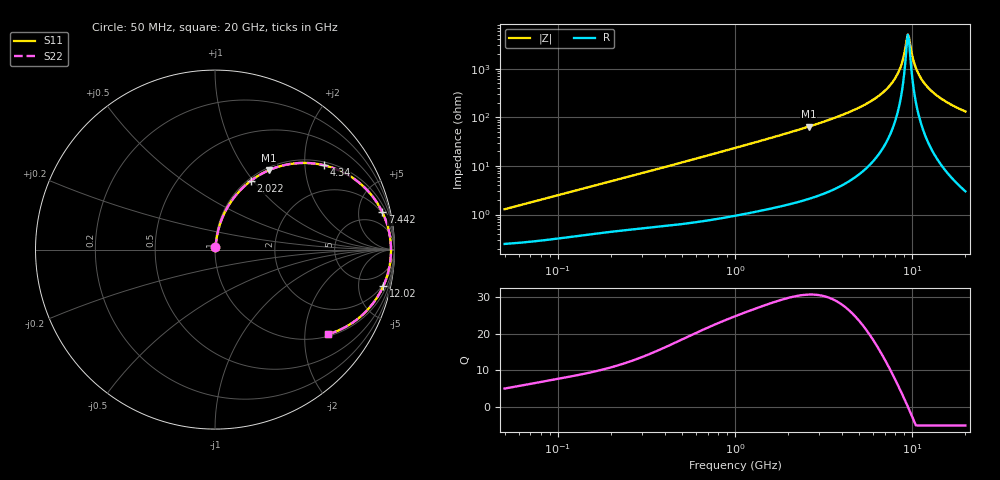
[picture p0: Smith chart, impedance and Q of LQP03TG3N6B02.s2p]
!Murata Part Number: LQP03TG3N6B02
!These Parameters are Measured in Series Mode Connection
!  o--[Z]--o
!Port1  Port2
!  o-------o
!Freq. Start=50[MHz] Stop=20[GHz], 401[Steps]
# Hz S RI R 50
!Freq.(Hz) S11(Real) S11(Imag) S21(Real) S21(Imag) S12(Real) S12(Imag) S22(Real) S22(Imag)
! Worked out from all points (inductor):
!   401 points, 50 MHz to 20 GHz, reference 50 ohm
!   read as one part in series: L = 4 nH near 51.52 MHz
!   highest Q = 30.7 at 2.608 GHz (marker M1), where L = 3.92 nH
!   self-resonance near 9.457 GHz
!   S11 on the Smith chart (normalised r, x): 50 MHz: 1.00, +0.03; 2.022 GHz: 1.03, +0.97; 4.34 GHz: 1.09, +2.49; 7.442 GHz: 1.82, +8.70; 12.02 GHz: 1.75, -8.95; 20 GHz: 1.06, -2.63
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5e7  0.00264 0.0126  0.9974 -0.0126  0.9974 -0.0126  0.00264 0.0126
1.364002e8  0.00481 0.0331  0.9952 -0.0331  0.9952 -0.0331  0.00481 0.0331
3.721004e8  0.0131 0.0861  0.9869 -0.0861  0.9869 -0.0861  0.0131 0.0861
1e9  0.0597 0.2177  0.9403 -0.2177  0.9403 -0.2177  0.0597 0.2177
2.021818e9  0.198 0.3821  0.802 -0.3821  0.802 -0.3821  0.198 0.3821
2.608132e9  0.2987 0.4417  0.7013 -0.4417  0.7013 -0.4417  0.2987 0.4417
2.728004e9  0.3202 0.4506  0.6798 -0.4506  0.6798 -0.4506  0.3202 0.4506
4.34015e9  0.6047 0.4705  0.3953 -0.4705  0.3953 -0.4705  0.6047 0.4705
5.944466e9  0.8185 0.3597  0.1815 -0.3597  0.1815 -0.3597  0.8185 0.3597
7.442007e9  0.9327 0.208  0.0673 -0.208  0.0673 -0.208  0.9327 0.208
8.020766e9  0.9571 0.1469  0.0429 -0.1469  0.0429 -0.1469  0.9571 0.1469
8.516016e9  0.9707 0.0956  0.0293 -0.0956  0.0293 -0.0956  0.9707 0.0956
8.907419e9  0.9772 0.0561  0.0228 -0.0561  0.0228 -0.0561  0.9772 0.0561
9.316812e9  0.9804 0.0162  0.0196 -0.0162  0.0196 -0.0162  0.9804 0.0162
9.457416e9  0.9808 0.00278  0.0192 -0.00278  0.0192 -0.00278  0.9808 0.00278
9.745021e9  0.9803 -0.024  0.0197 0.024  0.0197 0.024  0.9803 -0.024
1.019291e10  0.977 -0.064  0.023 0.064  0.023 0.064  0.977 -0.064
1.066139e10  0.9703 -0.1035  0.0297 0.1035  0.0297 0.1035  0.9703 -0.1035
1.131968e10  0.9565 -0.155  0.0435 0.155  0.0435 0.155  0.9565 -0.155
1.201863e10  0.9373 -0.2043  0.0627 0.2043  0.0627 0.2043  0.9373 -0.2043
1.482269e10  0.8344 -0.3515  0.1656 0.3515  0.1656 0.3515  0.8344 -0.3515
2e10  0.6312 -0.4712  0.3688 0.4712  0.3688 0.4712  0.6312 -0.4712
